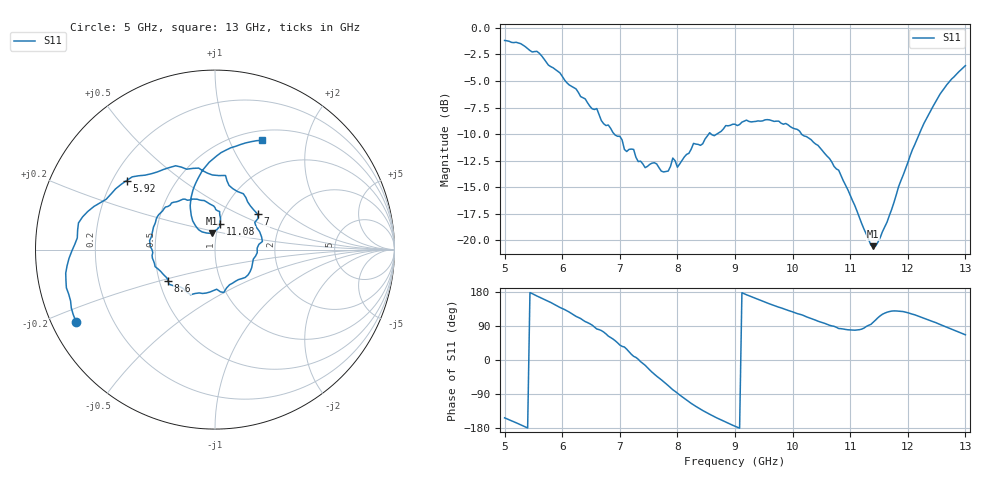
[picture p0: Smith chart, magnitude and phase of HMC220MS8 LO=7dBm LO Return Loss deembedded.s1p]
!Hittite Microwave Corporation
!12 Elizabeth Drive
!Chelmsford, MA 01824
!Tel: 978-250-3343
!Fax: 978-250-3373
!Device: HMC220MS8, 5-12 GHz, GaAS MMIC SMT Double-Balanced Mixer in 8-lead MSOP package
!Misc: LO power level=7dBm, Room
# MHZ S MA R 50
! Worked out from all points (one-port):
!   201 points, 5 GHz to 13 GHz, reference 50 ohm
!   lowest |S11| = -20.5 dB at 11.4 GHz (marker M1), VSWR 1.21, Z = 47.6 + j8.91 ohm
!   |S11| at or under -10 dB: 6.906 GHz to 8.543 GHz (1.637 GHz wide, 21.2 % of centre); 8.587 GHz to 8.682 GHz (94.66 MHz wide, 1.1 % of centre); 10.16 GHz to 12.2 GHz (2.042 GHz wide, 18.3 % of centre)
!   S11 on the Smith chart (normalised r, x): 5 GHz: 0.07, -0.24; 5.92 GHz: 0.26, +0.32; 7 GHz: 1.46, +0.64; 8.6 GHz: 0.56, -0.21; 11.08 GHz: 1.02, +0.30; 13 GHz: 0.61, +1.34
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5000  0.872 -152.6
5280  0.842 -171.0
5560  0.775 169.0
5920  0.625 142.0
6000  0.592 136.0
6240  0.516 115.2
6600  0.417 81.9
7000  0.309 39.5
7080  0.268 34.3
7240  0.268 9.7
7440  0.22 -13.9
7600  0.232 -37.5
7840  0.212 -67.4
7920  0.244 -78.5
8000  0.221 -87.6
8280  0.286 -118.5
8600  0.314 -146.3
9000  0.352 -174.7
9520  0.369 152.6
10000  0.338 127.0
10640  0.243 91.7
11000  0.163 79.3
11080  0.146 78.7
11400  0.094 99.6
11640  0.122 126.1
12000  0.232 124.8
12480  0.447 99.0
13000  0.664 66.5
